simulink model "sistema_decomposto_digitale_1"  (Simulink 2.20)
settings: Solver=VariableStepDiscrete  StartTime=0.0  StopTime=10.0  RelTol=1e-3  AbsTol=1e-6
undefined symbols (not defined in the file or in its folder): T

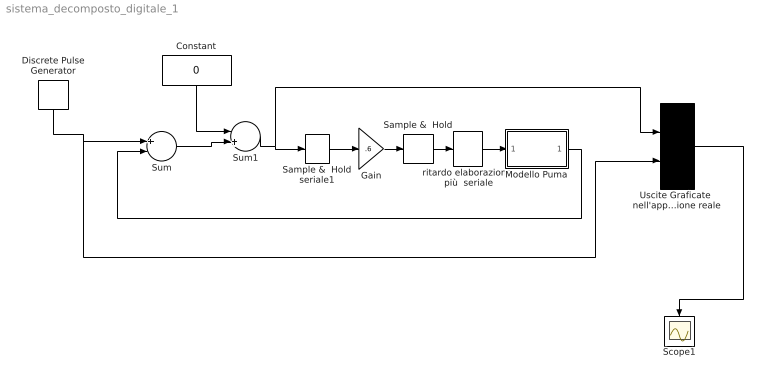
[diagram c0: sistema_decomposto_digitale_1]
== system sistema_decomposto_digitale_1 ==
  Constant : Constant  Orientation=down  Value=0
  Discrete Pulse Generator : DiscretePulseGenerator  Orientation=down  Amplitude=47  Period=100  PulseWidth=100  PhaseDelay=10  SampleTime=.1
  Gain : Gain  Gain=.6
  Modello Puma : Subsystem  Description=Modello Puma
  Sample &  Hold : ZeroOrderHold  SampleTime=.260
  Sample &  Hold seriale1 : ZeroOrderHold  SampleTime=T
  Scope1 : Scope
  Sum : Sum  Inputs=+-
  Sum1 : Sum  Inputs=-+
  Uscite Graficate  nell'applicazione reale : Mux  Inputs=2
  ritardo elaborazione  più  seriale : DiscreteTransferFcn  Numerator=1  Denominator=[1 0 0 0 0 0 0 0 0]  SampleTime=.032
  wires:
  Uscite Graficate  nell'applicazione reale/1 -> Scope1/1
  Sum/1 -> Sum1/2
  Discrete Pulse Generator/1 -> Sum/1, Uscite Graficate  nell'applicazione reale/2
  Constant/1 -> Sum1/1
  Gain/1 -> Sample &  Hold/1
  Sum1/1 -> Uscite Graficate  nell'applicazione reale/1, Sample &  Hold seriale1/1
  Modello Puma/1(Out1) -> Sum/2
  ritardo elaborazione  più  seriale/1 -> Modello Puma/1(In1)
  Sample &  Hold/1 -> ritardo elaborazione  più  seriale/1
  Sample &  Hold seriale1/1 -> Gain/1

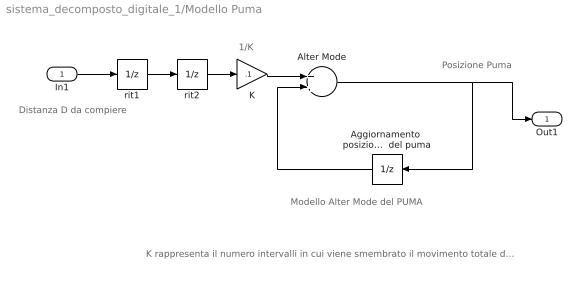
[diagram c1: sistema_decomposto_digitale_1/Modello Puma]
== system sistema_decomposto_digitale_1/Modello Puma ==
  note: Posizione Puma
  note: Modello Alter Mode del PUMA
  note: 1/K
  note: K rappresenta il numero intervalli in cui viene smembrato il movimento totale da compiere, dopo K time-slice (del PUMA) si ottiene che si e' compiuto proprio la distanza D trasmessa.
  note: Distanza D da compiere
  In1 : Inport  Port=1  PortWidth=-1  SampleTime=-1
  Aggiornamento  posizione   Il sample-time di questo blocco rappresenta la TIME-SLICE  del puma : UnitDelay  Orientation=left  X0=0  SampleTime=.032
  Alter Mode : Sum  Inputs=++
  K : Gain  Gain=.1
  rit1 : UnitDelay  X0=0  SampleTime=.032
  rit2 : UnitDelay  X0=0  SampleTime=.032
  Out1 : Outport  Port=1
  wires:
  K/1 -> Alter Mode/1
  Aggiornamento  posizione   Il sample-time di questo blocco rappresenta la TIME-SLICE  del puma/1 -> Alter Mode/2
  Alter Mode/1 -> Out1/1, Aggiornamento  posizione   Il sample-time di questo blocco rappresenta la TIME-SLICE  del puma/1
  In1/1 -> rit1/1
  rit1/1 -> rit2/1
  rit2/1 -> K/1
